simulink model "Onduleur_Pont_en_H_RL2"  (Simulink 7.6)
settings: Solver=ode15s  StartTime=0.0  StopTime=30  RelTol=1e-3
InitFcn:
  | clc
  | clear all
StopFcn:
  | close all, clc
  | load Vitesse_Consigne_position.mat
  | plot(x(1,:),x(2,:),x(1,:),x(3,:),x(1,:),x(4,:))
  | xlabel('temps')
  | title('Consigne et vitesse de rotation')
  | grid
  | 
  | load Cde_Position.mat
  | figure
  | plot(y(1,:),y(2,:),y(1,:),y(3,:))
  | xlabel('temps')
  | title('Signal de commande PID')
  | grid
  | 
  | delete *.mat
undefined symbols (not defined in the file or in its folder): blocks, Continuous, powergui, Ts, ZData
libraries: powerlib x14, fl_lib x12, nesl_utility x6, elec_lib x1, powerlib_extras x1

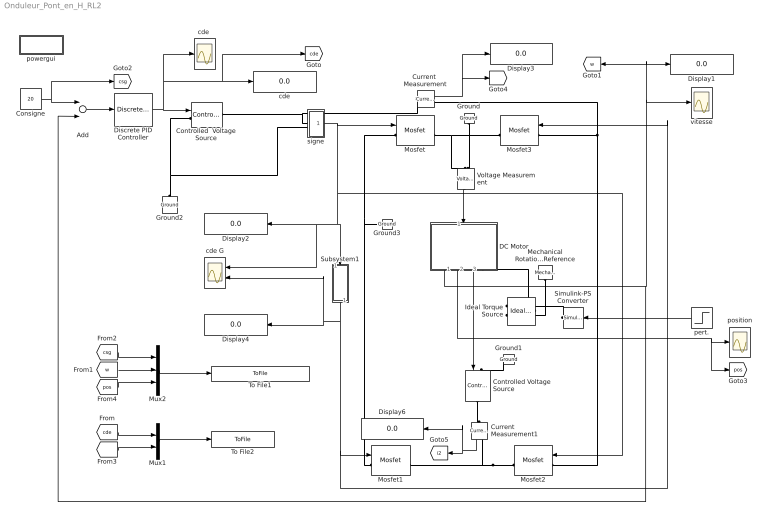
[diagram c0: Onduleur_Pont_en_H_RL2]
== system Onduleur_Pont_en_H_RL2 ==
  Add : Sum  Inputs=+-
  Consigne : Constant  Value=20
  Controlled  Voltage Source : powerlib/Electrical Sources/Controlled Voltage Source  DialogController=POWERSYS.PowerSysDialog  SystemSampleTime=-1  Initialize=on  Source_Type=AC  Amplitude=0  Phase=0  Frequency=0  Measurements=None
  Controlled Voltage Source : powerlib/Electrical Sources/Controlled Voltage Source  DialogController=POWERSYS.PowerSysDialog  SystemSampleTime=-1  Initialize=on  Source_Type=AC  Amplitude=0  Phase=0  Frequency=0  Measurements=None
  Current  Measurement : powerlib/Measurements/Current Measurement  DialogController=POWERSYS.PowerSysDialog  SystemSampleTime=-1  PhasorSimulation=off  OutputType=Complex  PSBequivalent=0
  Current  Measurement1 : powerlib/Measurements/Current Measurement  DialogController=POWERSYS.PowerSysDialog  SystemSampleTime=-1  PhasorSimulation=off  OutputType=Complex  PSBequivalent=0
  DC Motor : Subsystem
  Discrete PID Controller : powerlib_extras/Discrete  Control Blocks/Discrete PID Controller  DialogController=POWERSYS.PowerSysDialog  SystemSampleTime=-1  Kp=12  Ki=2  Kd=0  TcD=0  Par_Limits=[100 -100]  Init=0  Ts=5e-5
  Display{1..4,6} (5 alike) : Display
  Ground{,1..3} (4 alike) : powerlib/Elements/Ground  DialogController=POWERSYS.PowerSysDialog  PhysicalDomain=powersysdomain  SubClassName=unknown  LeftPortType=p1  RightPortType=p1  LConnTagsString=a
  Ideal Torque Source : fl_lib/Mechanical/Mechanical Sources/Ideal Torque Source  DialogController=NetworkEngine.DynNeDlgSource  SystemSampleTime=-1  w_Log=off  t_Log=off  LocalVarNames=|w|t  LocalVarDescs=|w|t  LocalVarLogging=[0 0]
  Mechanical Rotational Reference : fl_lib/Mechanical/Rotational Elements/Mechanical Rotational Reference  DialogController=NetworkEngine.DynNeDlgSource  SystemSampleTime=-1  t_Log=off  LocalVarNames=|t  LocalVarDescs=|t  LocalVarLogging=0
  Mosfet{,1..3} (4 alike) : powerlib/Power Electronics/Mosfet  DialogController=POWERSYS.PowerSysDialog  SystemSampleTime=-1  Ron=1e-6  Lon=0  Rd=0.001  Vfd=0  IC=0  Rs=1e8  Cs=inf  Measurements=on
  Mux1 : Mux  Inputs=2
  Mux2 : Mux  Inputs=3
  Simulink-PS Converter : nesl_utility/Simulink-PS Converter  DialogController=NetworkEngine.DynNeUtilDlgSource  SystemSampleTime=-1  PhysicalDomain=network_engine_domain  LeftPortType=input  RightPortType=output  SubClassName=ps_input  Unit=1  AffineConversion=off  InputFilterTimeConstant=.001  UdotUserProvided=0
  Subsystem1 : Subsystem
  To File1 : ToFile  Filename=Vitesse_Consigne_position  MatrixName=x
  To File2 : ToFile  Filename=Cde_Position  MatrixName=y
  Voltage Measurement : powerlib/Measurements/Voltage Measurement  DialogController=POWERSYS.PowerSysDialog  SystemSampleTime=-1  PhasorSimulation=off  OutputType=Complex  PSBequivalent=0
  cde : Display
  "cde " : Scope
  cde G : Scope  NumInputPorts=2
  pert. : Step  Time=25  Before=-0.001  After=0  SampleTime=0
  position : Scope
  powergui : Subsystem  AncestorBlock=powerlib/powergui  InitFcn=powergui( 'InitFcn_Callback' , gcb , 0 , [ ] );  StopFcn=powergui( 'StopFcn_Callback' , gcb , 0 , [ ] );  mask(PSB option menu block){SimulationMode=Continuous, SampleTime=Ts, frequency=60, SPID=off, DisableSnubberDevices=off, DisableRonSwitches=off, DisableVfSwitches=off, SwTol=0, Interpol=off, frequencyindice=0, echomessages=off, HookPort=off, DisplayEquations=off, FunctionMessages=off, EnableUseOfTLC=off, x0status=blocks, RestoreLinks=warning, ResistiveCurrentMeasurement=off, Frange=[0:2:500], Ylog=off, Xlog=on, ShowGrid=off, save=off, variable=ZData, structure=, ZoomFFT=on, StartTime=0.0, cycles=1, DisplayStyle=1, fundamental=60, FreqAxis=off, MaxFrequency=1000, frequencyindicesteady=1, RmsSteady=1, display=off, Ts=0, methode=off}
      mask prompts: SimulationMode "Simulation type:"; SampleTime "Sample time (s):"; frequency "Phasor frequency (Hz):"; SPID "Enable use of ideal switching devices"; DisableSnubberDevices "Disable snubbers in switching devices"; DisableRonSwitches "Disable On resistance in switching devices (Ron=0)"; DisableVfSwitches "Disable Forward voltage in switching devices (Vf=0)"; SwTol "Switch tolerance"; Interpol "Interpolate"; frequencyindice "Load flow frequency (Hz):"; echomessages "Display SimPowerSystems warnings and messages"; HookPort "Add a hook port to the powergui block"; DisplayEquations "Display circuit differential equations"; FunctionMessages "Display internal function messages (debug mode feature)"; EnableUseOfTLC "Use TLC file when in Accelerator Simulation Mode and for RTW applications"; x0status "Start simulation with initial electrical states from:"; RestoreLinks "Restore disabled links of SimPowerSystems blocks:"; ResistiveCurrentMeasurement "Use non ideal current measurement blocks (1e-4Ohm internal resistance)"; Frange "Frequency Range"; Ylog "Log impedance"; Xlog "log Frequency"; ShowGrid "grid"; save "Save Data To Workspace"; variable "Variable Name"; structure "Structure Name (PSBFFTSCOPE)"; ZoomFFT "ZoomFFT (PSBFFTSCOPE)"; StartTime "Start Time (PSBFFTSCOPE)"; cycles "Cycles (PSBFFTSCOPE)"; DisplayStyle "Display style (PSBFFTSCOPE)"; fundamental "Fundamental (PSBFFTSCOPE)"; FreqAxis "Frequency Axis (PSBFFTSCOPE)"; MaxFrequency "Max Frequency (PSBFFTSCOPE)"; frequencyindicesteady "Frequency indice (STEADYSTATE)"; RmsSteady "RMS display (STEADYSTATE)"; display "Display Results"; Ts "Old Ts setting (OBSOLETE)"; methode "Phasor simulation (OBSOLETE)"
      mask help: Set simulation type, simulation parameters, and preferences
      mask init:
      | message = powergui('MaskInitialization',gcb,SimulationMode,SampleTime);
  signe : Subsystem
  vitesse : Scope
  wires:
  Subsystem1/1(1-2u) -> Mosfet1/1, Mosfet3/1, Display4/1, cde G/2
  Voltage Measurement/1 -> DC Motor/1(U+)
  DC Motor/2(alpha) -> position/1, [pos]
  Add/1 -> Discrete PID Controller/1
  Consigne/1 -> [csg], Add/1
  signe/1(sgn) -> Mosfet2/1, Subsystem1/1(u), Display2/1, cde G/1, Mosfet/1
  DC Motor/1(w) -> Add/2, vitesse/1, [w], Display1/1
  Discrete PID Controller/1 -> Controlled  Voltage Source/1, "cde "/1, cde/1, [cde]
  pert./1 -> Simulink-PS Converter/1
  [w] -> Mux2/2
  Mux2/1 -> To File1/1
  [csg] -> Mux2/1
  [pos] -> Mux2/3
  Current  Measurement/1 -> [i], Display3/1
  [cde] -> Mux1/1
  [i] -> Mux1/2
  Mux1/1 -> To File2/1
  DC Motor/3(U-) -> Controlled Voltage Source/1
  Current  Measurement1/1 -> [i2], Display6/1
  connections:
  Mosfet2/RConn1 -- Mosfet1/RConn1 -- Current  Measurement1/RConn1
  Mosfet/RConn1 -- Mosfet3/RConn1 -- Voltage Measurement/LConn1
  Ground/LConn1 -- Voltage Measurement/LConn2
  Ground1/LConn1 -- Controlled Voltage Source/LConn1
  Mosfet1/LConn1 -- Mosfet/LConn1 -- Ground3/LConn1
  Ideal Torque Source/LConn1 -- DC Motor/RConn1
  Simulink-PS Converter/RConn1 -- Ideal Torque Source/RConn1
  Mosfet2/LConn1 -- Mosfet3/LConn1 -- Current  Measurement/RConn1
  Mechanical Rotational Reference/LConn1 -- Ideal Torque Source/RConn2
  signe/LConn1 -- Controlled  Voltage Source/RConn1 -- Current  Measurement/LConn1
  Controlled Voltage Source/RConn1 -- Current  Measurement1/LConn1
  Ground2/LConn1 -- Controlled  Voltage Source/LConn1 -- signe/LConn2

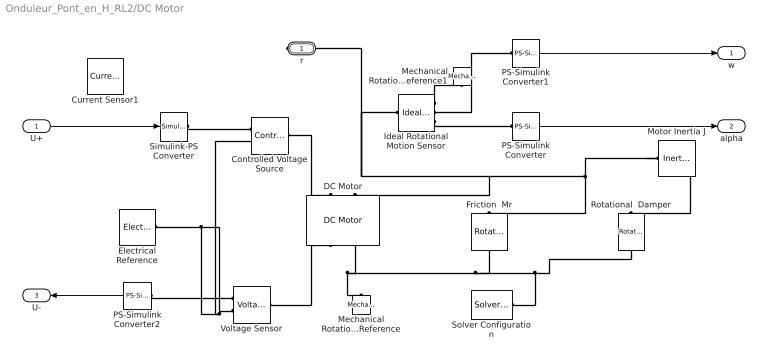
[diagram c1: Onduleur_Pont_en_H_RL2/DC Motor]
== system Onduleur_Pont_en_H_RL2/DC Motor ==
  U+ : Inport
  Controlled Voltage Source : fl_lib/Electrical/Electrical Sources/Controlled Voltage Source  DialogController=NetworkEngine.DynNeDlgSource  SystemSampleTime=-1  i_Log=off  v_Log=off  LocalVarNames=|i|v  LocalVarDescs=|i|v  LocalVarLogging=[0 0]
  Current Sensor1 : fl_lib/Electrical/Electrical Sensors/Current Sensor  DialogController=NetworkEngine.DynNeDlgSource  SystemSampleTime=-1  i1_Log=off  v1_Log=off  LocalVarNames=|i1|v1  LocalVarDescs=|i1|v1  LocalVarLogging=[0 0]
  DC Motor : elec_lib/Actuators & Drivers/Rotational Actuators/DC Motor  DialogController=NetworkEngine.DynNeDlgSource  SystemSampleTime=-1  parameterization=1  Ra=3.9 Ohm  La=1.2e-3 H  emf_or_torque=2  Kv=7.2e-5 V/rpm  Ki=10e-3 N*m/A  T_stall=2.4e-4 N*m  w_max=1.91e+4 rpm  w_rated=1.5e+4 rpm  P_rated=0.08 W  V_rated=1.5 V  J=0.01 g*cm^2  lam=1e-8 N*m/(rad/s)  speed0=0 rpm  current_Log=off  voltage_Log=off  power_Log=off  i2r_Log=off  torque_Log=off  speed_Log=off  LocalVarNames=|current|voltage|power|i2r|torque|speed  LocalVarDescs=|Current (A)|Voltage (V)|Power (W)|Electrical losses (W)|Torque (Nm)|Angular speed (rad/s)  LocalVarLogging=[0 0 0 0 0 0]
  Electrical Reference : fl_lib/Electrical/Electrical Elements/Electrical Reference  DialogController=NetworkEngine.DynNeDlgSource  SystemSampleTime=-1  i_Log=off  LocalVarNames=|i  LocalVarDescs=|i  LocalVarLogging=0
  Friction  Mr : fl_lib/Mechanical/Rotational Elements/Rotational Friction  DialogController=NetworkEngine.DynNeDlgSource  SystemSampleTime=-1  brkwy_trq=0.01e-3 N*m  Col_trq=0.01e-3 N*m  visc_coef=0.001e-3 N*m/(rad/s)  trans_coef=10 s/rad  vel_thr=0.1 rad/s  t_Log=off  w_Log=off  LocalVarNames=|friction_torque|rel_velocity|power  LocalVarDescs=|Friction torque (N*m)|Relative velocity (rad/s)|Power (W)  LocalVarLogging=[0 0 0]
  Ideal Rotational Motion Sensor : fl_lib/Mechanical/Mechanical Sensors/Ideal Rotational Motion Sensor  DialogController=NetworkEngine.DynNeDlgSource  SystemSampleTime=-1  offset=0 rad  w_Log=off  t_Log=off  phi_Log=off  LocalVarNames=|w|t|phi  LocalVarDescs=|w|t|phi  LocalVarLogging=[0 0 0]
  Mechanical Rotational Reference : fl_lib/Mechanical/Rotational Elements/Mechanical Rotational Reference  DialogController=NetworkEngine.DynNeDlgSource  SystemSampleTime=-1  t_Log=off  LocalVarNames=|t  LocalVarDescs=|t  LocalVarLogging=0
  Mechanical Rotational Reference1 : fl_lib/Mechanical/Rotational Elements/Mechanical Rotational Reference  DialogController=NetworkEngine.DynNeDlgSource  SystemSampleTime=-1  t_Log=off  LocalVarNames=|t  LocalVarDescs=|t  LocalVarLogging=0
  Motor Inertia J : fl_lib/Mechanical/Rotational Elements/Inertia  DialogController=NetworkEngine.DynNeDlgSource  SystemSampleTime=-1  inertia=0.001 g*cm^2  initial_velocity=0 rad/s  t_Log=off  LocalVarNames=|torque|velocity  LocalVarDescs=|Inertia torque (N*m)|Inertia absolute velocity (rad/s)  LocalVarLogging=[0 0]
  PS-Simulink Converter : nesl_utility/PS-Simulink Converter  DialogController=NetworkEngine.DynNeUtilDlgSource  SystemSampleTime=-1  PhysicalDomain=network_engine_domain  LeftPortType=input  RightPortType=output  SubClassName=ps_output  Unit=1  AffineConversion=off
  PS-Simulink Converter1 : nesl_utility/PS-Simulink Converter  DialogController=NetworkEngine.DynNeUtilDlgSource  SystemSampleTime=-1  PhysicalDomain=network_engine_domain  LeftPortType=input  RightPortType=output  SubClassName=ps_output  Unit=1  AffineConversion=off
  PS-Simulink Converter2 : nesl_utility/PS-Simulink Converter  DialogController=NetworkEngine.DynNeUtilDlgSource  SystemSampleTime=-1  PhysicalDomain=network_engine_domain  LeftPortType=input  RightPortType=output  SubClassName=ps_output  Unit=1  AffineConversion=on
  Rotational  Damper : fl_lib/Mechanical/Rotational Elements/Rotational Damper  DialogController=NetworkEngine.DynNeDlgSource  SystemSampleTime=-1  D=0.001 N*m/(rad/s)  t_Log=off  w_Log=off  LocalVarNames=|t|w  LocalVarDescs=|t|w  LocalVarLogging=[0 0]
  Simulink-PS Converter : nesl_utility/Simulink-PS Converter  DialogController=NetworkEngine.DynNeUtilDlgSource  SystemSampleTime=-1  PhysicalDomain=network_engine_domain  LeftPortType=input  RightPortType=output  SubClassName=ps_input  Unit=1  AffineConversion=off  InputFilterTimeConstant=.001  UdotUserProvided=0
  Solver Configuration : nesl_utility/Solver Configuration  DialogController=NetworkEngine.DynNeUtilDlgSource  SystemSampleTime=-1  PhysicalDomain=network_engine_domain  LeftPortType=input  RightPortType=generic  SubClassName=solver  Accelerate=off  Profile=off  ResidualTolerance=1e-9  MaxNonlinIter=3  MaxModeIter=2  DoFixedCost=off  UseLocalSampling=off  DoDC=off  LinearAlgebra=Sparse  LocalSolverSampleTime=.001  LocalSolverChoice=NE_BACKWARD_EULER_ADVANCER  UseLocalSolver=off
  Voltage Sensor : fl_lib/Electrical/Electrical Sensors/Voltage Sensor  DialogController=NetworkEngine.DynNeDlgSource  SystemSampleTime=-1  i1_Log=off  v1_Log=off  LocalVarNames=|i1|v1  LocalVarDescs=|i1|v1  LocalVarLogging=[0 0]
  r : PMIOPort  Port=1  Side=Right
  w : Outport
  alpha : Outport  Port=2
  U- : Outport  Port=3
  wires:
  U+/1 -> Simulink-PS Converter/1
  PS-Simulink Converter/1 -> alpha/1
  PS-Simulink Converter1/1 -> w/1
  PS-Simulink Converter2/1 -> U-/1
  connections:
  Ideal Rotational Motion Sensor/RConn3 -- PS-Simulink Converter/LConn1
  Ideal Rotational Motion Sensor/RConn2 -- PS-Simulink Converter1/LConn1
  Ideal Rotational Motion Sensor/RConn1 -- Mechanical Rotational Reference1/LConn1
  Solver Configuration/RConn1 -- Rotational  Damper/RConn1 -- Friction  Mr/RConn1 -- DC Motor/RConn2 -- Mechanical Rotational Reference/LConn1
  Motor Inertia J/LConn1 -- Rotational  Damper/LConn1 -- Friction  Mr/LConn1 -- DC Motor/LConn2 -- r/RConn1 -- Ideal Rotational Motion Sensor/LConn1
  PS-Simulink Converter2/LConn1 -- Voltage Sensor/RConn1
  Voltage Sensor/LConn1 -- DC Motor/RConn1
  Voltage Sensor/RConn2 -- Controlled Voltage Source/RConn2 -- Electrical Reference/LConn1
  Simulink-PS Converter/RConn1 -- Controlled Voltage Source/RConn1
  Controlled Voltage Source/LConn1 -- DC Motor/LConn1

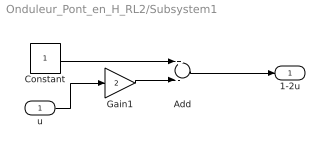
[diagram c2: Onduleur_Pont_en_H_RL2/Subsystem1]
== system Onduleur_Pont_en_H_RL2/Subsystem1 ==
  u : Inport
  Add : Sum  Inputs=+-
  Constant : Constant
  Gain1 : Gain  Gain=2
  1-2u : Outport
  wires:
  u/1 -> Gain1/1
  Add/1 -> 1-2u/1
  Constant/1 -> Add/1
  Gain1/1 -> Add/2

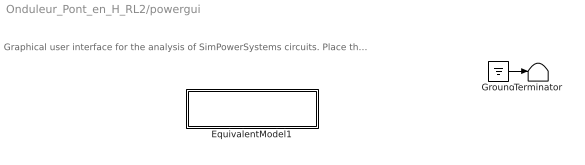
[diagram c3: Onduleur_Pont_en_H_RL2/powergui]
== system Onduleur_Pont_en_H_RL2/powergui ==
  note: Graphical user interface for the analysis of SimPowerSystems circuits. Place the Powergui block in the top-level of your model and double-click on it to open the GUI.
  EquivalentModel1 : Subsystem
  Ground : Ground
  Terminator : Terminator
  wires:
  Ground/1 -> Terminator/1

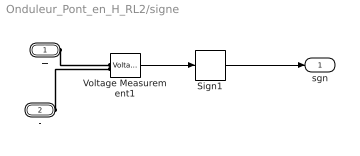
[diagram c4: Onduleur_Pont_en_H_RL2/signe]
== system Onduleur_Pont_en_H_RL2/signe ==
  Sign1 : Signum
  Voltage Measurement1 : powerlib/Measurements/Voltage Measurement  DialogController=POWERSYS.PowerSysDialog  SystemSampleTime=-1  PhasorSimulation=off  OutputType=Complex  PSBequivalent=0
  + : PMIOPort  Port=1  Side=Left
  - : PMIOPort  Port=2  Side=Left
  sgn : Outport
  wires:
  Voltage Measurement1/1 -> Sign1/1
  Sign1/1 -> sgn/1
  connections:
  +/RConn1 -- Voltage Measurement1/LConn1
  -/RConn1 -- Voltage Measurement1/LConn2

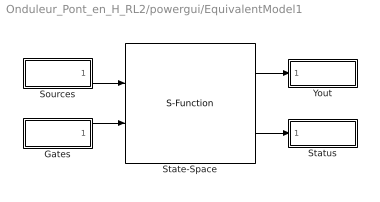
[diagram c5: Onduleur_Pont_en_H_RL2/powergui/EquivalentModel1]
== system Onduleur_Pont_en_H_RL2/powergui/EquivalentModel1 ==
  Gates : Subsystem
  Sources : Subsystem
  State-Space : S-Function  FunctionName=sfun_spssw_contc  Parameters=S.A, S.B, S.C, S.D, S.x0, S.EnableUseOfTLC,S.SwitchResistance ,S.SwitchType, S.SwitchGateInitialValue, S.OutputsToResetToZero  EnableBusSupport=off
  Status : Subsystem
  Yout : Subsystem
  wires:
  Gates/1(gates) -> State-Space/2
  Sources/1(u) -> State-Space/1
  State-Space/2 -> Status/1(status)
  State-Space/1 -> Yout/1(v,i)

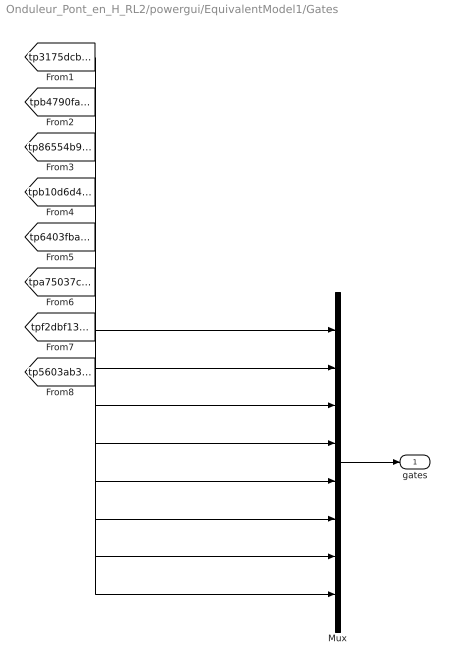
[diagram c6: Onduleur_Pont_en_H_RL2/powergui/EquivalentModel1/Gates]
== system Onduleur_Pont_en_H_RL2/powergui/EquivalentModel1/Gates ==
  Mux : Mux  Inputs=[1 1 1 1 1 1 1 1]
  gates : Outport
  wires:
  Mux/1 -> gates/1
  [tp3175dcb8_2fd4_4324_a5ed_0aea1fa5163c] -> Mux/1
  [tpb4790fa9_cb68_4d74_89be_c2a854522932] -> Mux/2
  [tp86554b9e_d017_4034_988c_db04acf0abb3] -> Mux/3
  [tpb10d6d49_69bb_4617_97ed_a18ea9136171] -> Mux/4
  [tp6403fba2_a464_487a_a64d_bbbf79ed9af5] -> Mux/5
  [tpa75037cb_5246_4dcf_8583_c228c2893df1] -> Mux/6
  [tpf2dbf137_a4cf_4397_bbd6_99c606be3fe2] -> Mux/7
  [tp5603ab39_1fb9_49fa_85e3_375b55811cfb] -> Mux/8

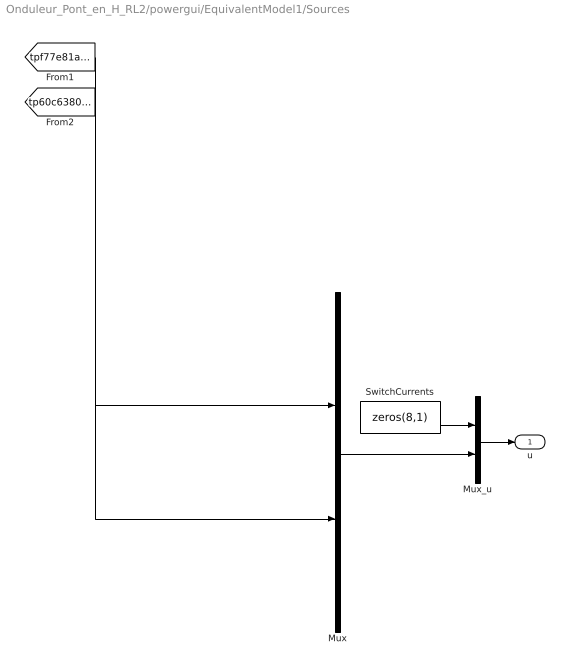
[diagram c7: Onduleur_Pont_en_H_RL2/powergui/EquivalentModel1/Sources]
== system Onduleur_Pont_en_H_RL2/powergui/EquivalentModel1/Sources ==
  Mux : Mux  Inputs=[1 1]
  Mux_u : Mux  Inputs=[8 2]
  SwitchCurrents : Constant  Value=zeros(8,1)
  u : Outport
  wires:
  Mux/1 -> Mux_u/2
  SwitchCurrents/1 -> Mux_u/1
  Mux_u/1 -> u/1
  [tpf77e81aa_a07d_4aa4_83d2_ecc7e8a0e2f5] -> Mux/1
  [tp60c6380b_289c_4881_ab49_1d7f701cdeda] -> Mux/2

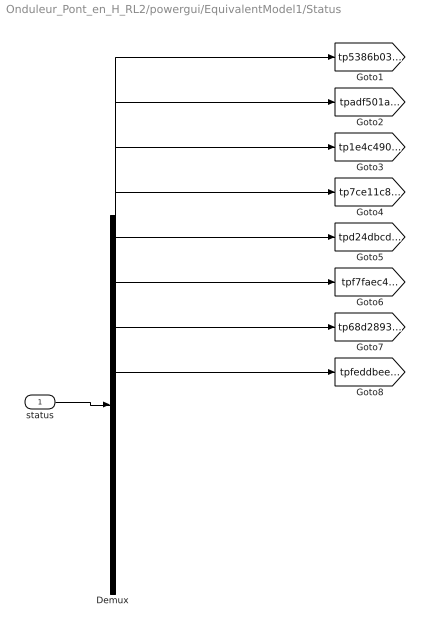
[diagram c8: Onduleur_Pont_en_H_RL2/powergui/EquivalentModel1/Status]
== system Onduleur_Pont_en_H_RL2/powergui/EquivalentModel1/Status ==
  status : Inport
  Demux : Demux  Outputs=[1 1 1 1 1 1 1 1]
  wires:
  status/1 -> Demux/1
  Demux/1 -> [tp5386b03d_8955_47b5_90bf_520c3025c4a0]
  Demux/2 -> [tpadf501ac_190d_40e7_8207_608bb6c8fcf2]
  Demux/3 -> [tp1e4c490b_9b36_4ac1_90a3_63d24ed29ec0]
  Demux/4 -> [tp7ce11c8b_e831_4163_8b4a_a7003e7cb854]
  Demux/5 -> [tpd24dbcd0_e35b_4de0_9ddd_c023955fb824]
  Demux/6 -> [tpf7faec49_5956_410b_b28a_7a61bf12e0ab]
  Demux/7 -> [tp68d2893b_06db_46ce_a2e0_aed70d3d0987]
  Demux/8 -> [tpfeddbeec_1d74_49f2_8bad_df33032bf7d2]

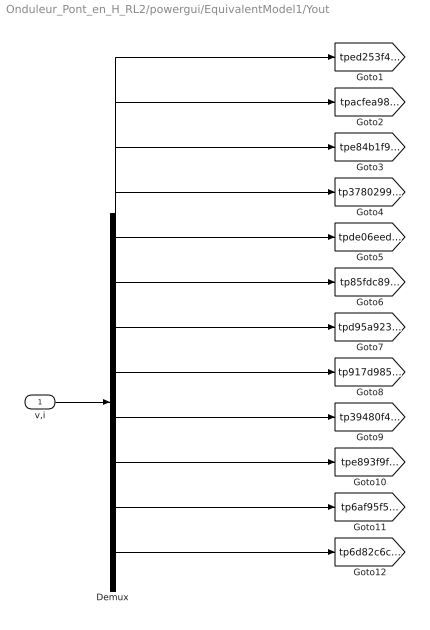
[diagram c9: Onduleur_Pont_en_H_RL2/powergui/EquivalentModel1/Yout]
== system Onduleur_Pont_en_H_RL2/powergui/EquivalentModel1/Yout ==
  v,i : Inport
  Demux : Demux  Outputs=[1 1 1 1 1 1 1 1 1 1 1 1]
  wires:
  v,i/1 -> Demux/1
  Demux/1 -> [tped253f4d_b607_4d6d_821f_66026cd86313]
  Demux/2 -> [tpacfea98d_3549_44f5_a4bc_07cfab1e0865]
  Demux/3 -> [tpe84b1f97_81a2_4dba_a78f_9be5bfdd8ae1]
  Demux/4 -> [tp37802998_89b5_454e_9f3d_064f7e5fdcd5]
  Demux/5 -> [tpde06eed5_b301_4983_a793_01c42fd0097d]
  Demux/6 -> [tp85fdc89a_d4b1_4d65_9bfe_462793152935]
  Demux/7 -> [tpd95a9237_c989_4d86_9e33_ee546f7477f3]
  Demux/8 -> [tp917d985b_c472_4962_858d_e62f607320e6]
  Demux/9 -> [tp39480f45_2491_4776_9017_8a5b8095acd0]
  Demux/10 -> [tpe893f9f4_7603_4075_85c6_210752fbf6e1]
  Demux/11 -> [tp6af95f53_c1bf_481a_8709_b2e2ff958e0f]
  Demux/12 -> [tp6d82c6ca_4c56_46f2_919f_768242dbaead]
